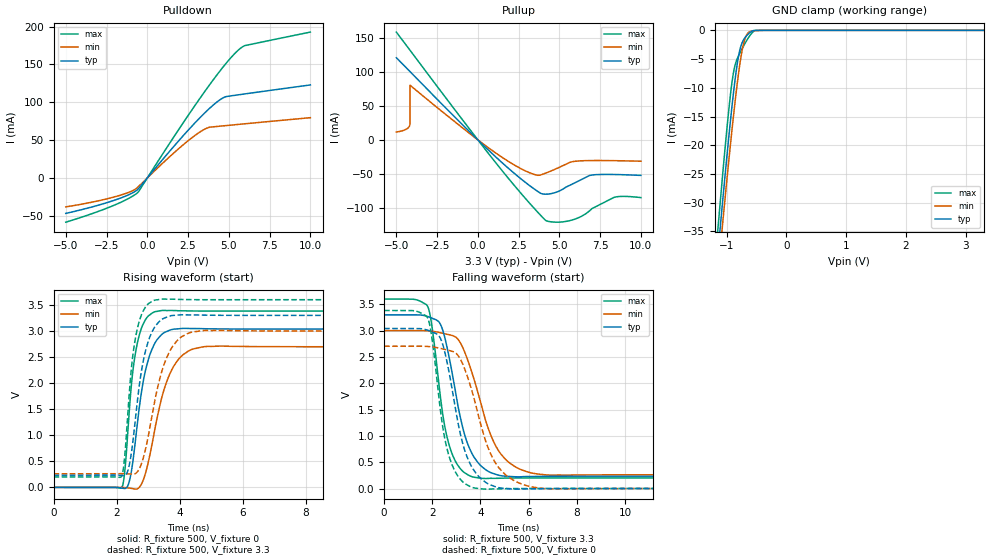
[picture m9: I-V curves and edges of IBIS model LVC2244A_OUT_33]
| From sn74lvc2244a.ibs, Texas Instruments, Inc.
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[Model]   LVC2244A_OUT_33
Model_type  3-state
Enable   Active-Low
Vref =   0
Rref =   500
Cref =   50p
Vmeas =   1.5
| variable   typ   min   max
C_comp   6.85pF   6.41pF   7.32pF
| C_pullup   5.73pF   5.15pF   6.77pF
| C_pulldown   5.38pF   4.98pF   5.63pF
| C_tri-state   6.85pF   6.41pF   7.32pF
[Temperature Range]   40   100   -40
| Ambient temperature   25   85   -40
[Voltage range]   3.3   3   3.6
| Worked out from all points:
|   slope of the pulldown table from 0 to 0.495 V, typ, clamps not added: 38.3 ohm
|   slope of the pullup table from 0 to 0.495 V, typ, clamps not added: 43 ohm
|   GND clamp passes 1 mA (typ) near -0.67 V on its own axis
|   rising waveform, R_fixture 500, V_fixture 0: 20-80 % time 457ps typ, 650ps min, 327ps max; typ from 0 V to 3.04 V
|   falling waveform, R_fixture 500, V_fixture 3.3: 20-80 % time 859ps typ, 1.17ns min, 632ps max; typ from 3.3 V to 0.234 V
|   rising waveform, R_fixture 500, V_fixture 3.3: 20-80 % time 439ps typ, 621ps min, 321ps max; typ from 0.234 V to 3.3 V
|   falling waveform, R_fixture 500, V_fixture 0: 20-80 % time 840ps typ, 1.12ns min, 628ps max; typ from 3.04 V to 0 V
[GND Clamp]
| LVC2244A_OUT_33
|   Voltage   I(typ)   I(min)   I(max)
-5V       -524.6mA   -512.3mA   -544.5mA
-1.145V   -38.63mA   -42.25mA   -34.43mA
-1.095V   -32.91mA   -36.71mA   -28.44mA
-1.075V   -30.65mA   -34.51mA   -26.09mA
-955mV    -17.65mA   -21.77mA   -12.96mA
-885mV    -10.83mA   -14.84mA   -7.323mA
-825mV    -5.994mA   -9.446mA   -4.992mA
-775mV    -3.247mA   -5.592mA   -3.878mA
-705mV    -1.448mA   -1.848mA   -2.501mA
-635mV    -604.2uA   -373uA     -1.27mA
-515mV    -15.29uA   -57.67uA   -13.6uA
3.3V      62.9pA     44.06nA    -1.528nA
[Pulldown]
| LVC2244A_OUT_33
|   Voltage   I(typ)   I(min)   I(max)
-5V       -46.84mA   -38.21mA   -58.44mA
-2.01V    -29.38mA   -24.99mA   -35.82mA
-1.055V   -21.35mA   -18.29mA   -25.97mA
-585mV    -15.13mA   -12.23mA   -19.25mA
1.805V    46.13mA    36.48mA    60.09mA
3.325V    81.74mA    62.09mA    108.2mA
3.81V     91.87mA    66.99mA    122.9mA
4.63V     105.7mA    68.82mA    146.2mA
5.25V     108.9mA    70.11mA    161.9mA
5.725V    110.3mA    71.09mA    171.6mA
6.025V    111.2mA    71.7mA     175.2mA
10V       123mA      79.69mA    192.8mA
[Pullup]
| LVC2244A_OUT_33
|   Voltage   I(typ)   I(min)   I(max)
-5V       121.1mA    11.55mA    158.8mA
-4.425V   107.1mA    15.3mA     140.5mA
-4.18V    101.1mA    21.38mA    132.6mA
-4.165V   100.7mA    23.51mA    132.2mA
-4.16V    100.6mA    80.49mA    132mA
1.665V    -37.47mA   -28.53mA   -50.6mA
3.38V     -71.02mA   -50.31mA   -98.87mA
4.15V     -80mA      -49mA      -118.5mA
5.625V    -67.02mA   -33.28mA   -119mA
6.935V    -52.01mA   -30.44mA   -102.7mA
8.425V    -51.04mA   -30.64mA   -84.24mA
10V       -52.34mA   -31.43mA   -84.99mA
[Ramp]
| LVC2244A_OUT_33
| variable   typ   min   max
dV/dt_r   1.84/4.73E-10   1.64/6.77E-10   2.04/3.33E-10
dV/dt_f   1.84/8.78E-10   1.65/1.20E-09   2.04/6.39E-10
R_load = 500
[Rising Waveform]
| LVC2244A_OUT_33
R_fixture =   500
C_fixture =   0
L_fixture =   0
V_fixture =   0
V_fixture_min = 0
V_fixture_max = 0
|   Time   V(typ)   V(min)   V(max)
0s        831.5pV    2.73nV     28.01nV
2.17ns    -13.75mV   -1.326mV   5.318mV
2.27ns    -21.2mV    -4.284mV   360.4mV
2.425ns   164mV      -14.99mV   1.627V
2.675ns   1.295V     -22.92mV   2.807V
2.995ns   2.42V      449.6mV    3.279V
3.425ns   2.927V     1.698V     3.392V
4ns       3.044V     2.481V     3.388V
4.895ns   3.042V     2.704V     3.381V
50ns      3.038V     2.699V     3.382V
[Falling Waveform]
| LVC2244A_OUT_33
R_fixture =   500
C_fixture =   0
L_fixture =   0
V_fixture =   3.3
V_fixture_min = 3
V_fixture_max = 3.6
|   Time   V(typ)   V(min)   V(max)
0s        3.3V       3V         3.6V
1.805ns   3.269V     2.996V     3.464V
2.3ns     3.15V      2.964V     1.884V
2.535ns   2.84V      2.939V     1.142V
2.835ns   2.169V     2.907V     644mV
3.305ns   1.085V     2.637V     311.6mV
3.76ns    578.1mV    2.036V     212.2mV
4.83ns    245mV      665.8mV    195.1mV
6.69ns    231.8mV    259.5mV    201.1mV
50ns      234.1mV    260.8mV    200.9mV
[Rising Waveform]
| LVC2244A_OUT_33
R_fixture =   500
C_fixture =   0
L_fixture =   0
V_fixture =   3.3
V_fixture_min = 3
V_fixture_max = 3.6
|   Time   V(typ)   V(min)   V(max)
0s        234mV      260.8mV    200.8mV
2.145ns   229.4mV    263.6mV    201.2mV
2.25ns    225.6mV    263.2mV    534.8mV
2.4ns     415.4mV    258.6mV    1.766V
2.66ns    1.644V     298.4mV    3.042V
2.95ns    2.685V     814.8mV    3.484V
3.41ns    3.209V     2.169V     3.609V
3.965ns   3.306V     2.84V      3.605V
4.84ns    3.303V     3.01V      3.599V
50ns      3.3V       3V         3.6V
[Falling Waveform]
| LVC2244A_OUT_33
R_fixture =   500
C_fixture =   0
L_fixture =   0
V_fixture =   0
V_fixture_min = 0
V_fixture_max = 0
|   Time   V(typ)   V(min)   V(max)
0s        3.04V      2.703V     3.383V
1.805ns   3.009V     2.699V     3.244V
1.99ns    2.975V     2.691V     2.842V
2.295ns   2.889V     2.667V     1.649V
2.835ns   1.857V     2.606V     435.7mV
3.285ns   820.3mV    2.342V     117mV
3.79ns    306mV      1.615V     6.291mV
4.755ns   16.9mV     398.6mV    -7.293mV
6.67ns    -2.48mV    -1.584mV   451uV
50ns      25.07uV    42.26uV    7.265uV
